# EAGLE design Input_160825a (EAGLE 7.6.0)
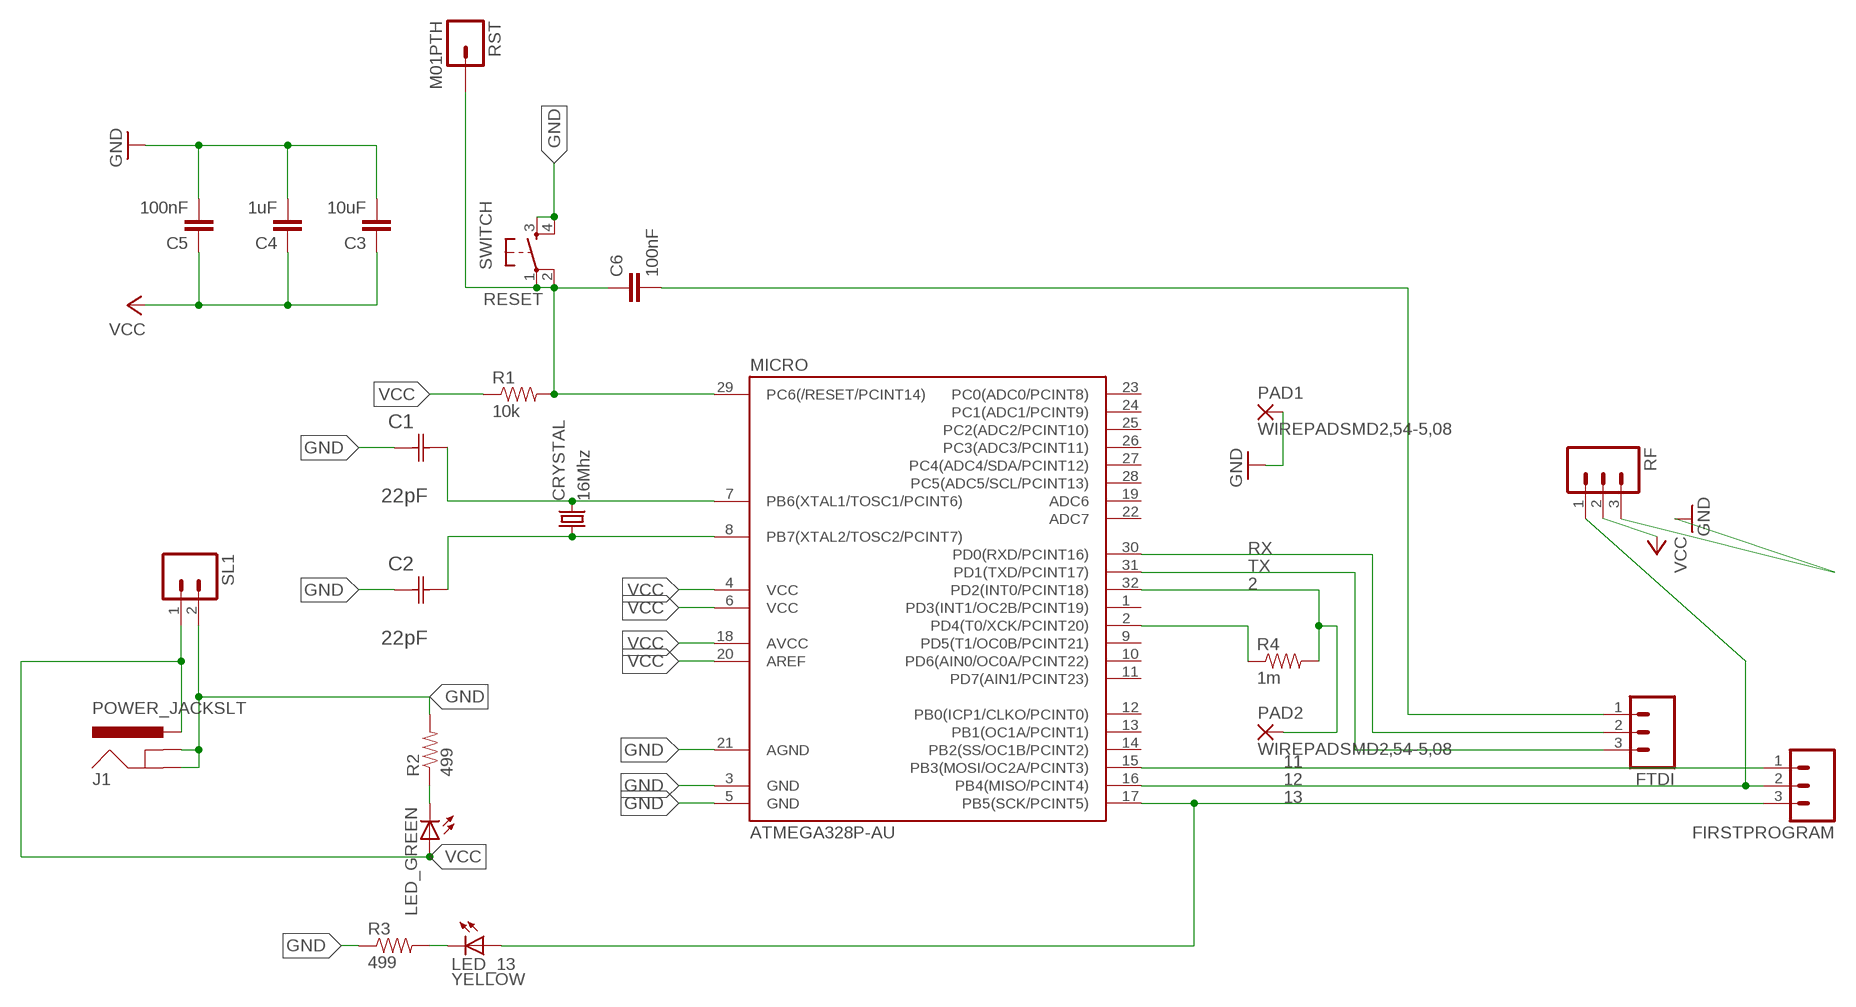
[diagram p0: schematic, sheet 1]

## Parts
C1  22pF  0612ZC225MAT2A  [CAPC3216X178N]
C2  22pF  0612ZC225MAT2A  [CAPC3216X178N]
C3  10uF  CAP1206  [1206]
C4  1uF  CAP1206  [1206]
C5  100nF  CAP1206  [1206]
C6  100nF  CAP1206  [1206]
CRYSTAL  16Mhz  CSM-7X-DU  [CSM-7X-DU]
FIRSTPROGRAM  M03  [03P]
FTDI  M03  [03P]
J1  POWER_JACKSLT  [POWER_JACK_SLOT]
LED_13  YELLOW  LED1206  [1206]
LED_GREEN  LED1206  [1206]
MICRO  ATMEGA328P-AU  ATMEGA48/88/168-AU  [TQFP32-08]
PAD1  WIREPADSMD2,54-5,08  [SMD2,54-5,08]
PAD2  WIREPADSMD2,54-5,08  [SMD2,54-5,08]
R1  10k  RESISTOR1206  [1206]
R2  499  RESISTOR1206  [1206]
R3  499  RESISTOR1206  [1206]
R4  1m  RESISTOR1206  [1206]
RF  M03  [03P]
RST  M01PTH  [1X01]
SL1  M02  [02P]
SWITCH  6MM_SWITCH6MM_SWITCH  [6MM_SWITCH]

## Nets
2: MICRO.32(PD2(INT0/PCINT18)) PAD2.1(P) R4.2
11: FIRSTPROGRAM.1 MICRO.15(PB3(MOSI/OC2A/PCINT3))
12: FIRSTPROGRAM.2 MICRO.16(PB4(MISO/PCINT4)) RF.1
13: FIRSTPROGRAM.3 LED_13.1(A) MICRO.17(PB5(SCK/PCINT5))
GND: C1.1(C1) C2.1(C1) C3.2 C4.2 C5.2 J1.GND@1(GNDBREAK) J1.GND@2(GND) MICRO.3(GND) MICRO.5(GND) MICRO.21(AGND) PAD1.1(P) R2.2 R3.1 RF.3 SL1.2 SWITCH.3(S) SWITCH.4(S1)
N$2: C1.2(C2) CRYSTAL.2 MICRO.7(PB6(XTAL1/TOSC1/PCINT6))
N$3: C6.2 FTDI.1
N$8: MICRO.2(PD4(T0/XCK/PCINT20)) R4.1
N$9: C2.2(C2) CRYSTAL.1 MICRO.8(PB7(XTAL2/TOSC2/PCINT7))
N$26: LED_GREEN.2(C) R2.1
N$27: LED_13.2(C) R3.2
RESET: C6.1 MICRO.29(PC6(/RESET/PCINT14)) R1.2 RST.1 SWITCH.1(P) SWITCH.2(P1)
RX: FTDI.2 MICRO.30(PD0(RXD/PCINT16))
TX: FTDI.3 MICRO.31(PD1(TXD/PCINT17))
VCC: C3.1 C4.1 C5.1 J1.PWR LED_GREEN.1(A) MICRO.4(VCC) MICRO.6(VCC) MICRO.18(AVCC) MICRO.20(AREF) R1.1 RF.2 SL1.1
Unconnected: MICRO.1(PD3(INT1/OC2B/PCINT19)) MICRO.9(PD5(T1/OC0B/PCINT21)) MICRO.10(PD6(AIN0/OC0A/PCINT22)) MICRO.11(PD7(AIN1/PCINT23)) MICRO.12(PB0(ICP1/CLKO/PCINT0)) MICRO.13(PB1(OC1A/PCINT1)) MICRO.14(PB2(SS/OC1B/PCINT2)) MICRO.19(ADC6) MICRO.22(ADC7) MICRO.23(PC0(ADC0/PCINT8)) MICRO.24(PC1(ADC1/PCINT9)) MICRO.25(PC2(ADC2/PCINT10)) MICRO.26(PC3(ADC3/PCINT11)) MICRO.27(PC4(ADC4/SDA/PCINT12)) MICRO.28(PC5(ADC5/SCL/PCINT13))

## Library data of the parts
C1 C2 = AVX_By_element14_Batch_1:0612ZC225MAT2A: Capacitor 1206; MPN: 0612ZC225MAT2A; OC_FARNELL: -; OC_NEWARK: 12N3209; SUPPLIER: AVX; TOLERANCE: ±20%; VALUE: 2.2µF; VOLTAGERATING: 10V
C3-C6 = 01_SparkFun:CAP: Capacitor
CRYSTAL = 01_FAB_Hello:CSM-7X-DU: SMD CRYSTAL; OC_FARNELL: unknown; OC_NEWARK: unknown
FIRSTPROGRAM FTDI RF = con-amp-quick:M03: AMP QUICK CONNECTOR; OC_FARNELL: unknown; OC_NEWARK: unknown
J1 = jib-fab:POWER_JACK: Power Jack This is the standard 5.5mm barrel jack for power. The PTH is the most common, proven, reliable, footprint. The Slot footprint only works if the mill layer is transmitted to the PCB fab house so be warned. Mating wall wart : TOL-00298 (and others); PROD_ID: PRT-00119
LED_13 LED_GREEN = 01_FAB_Hello:LED
MICRO = atmega8:ATMEGA48/88/168
PAD1 PAD2 = wirepad:WIREPAD: Wire PAD connect wire on PCB
R1-R4 = 01_SparkFun:RESISTOR: Resistor
RST = 01_SparkFun:M01: Header 1
SL1 = con-amp-quick:M02: AMP QUICK CONNECTOR; OC_FARNELL: unknown; OC_NEWARK: unknown
SWITCH = 01_FAB_Hello:6MM_SWITCH: OMRON SWITCH

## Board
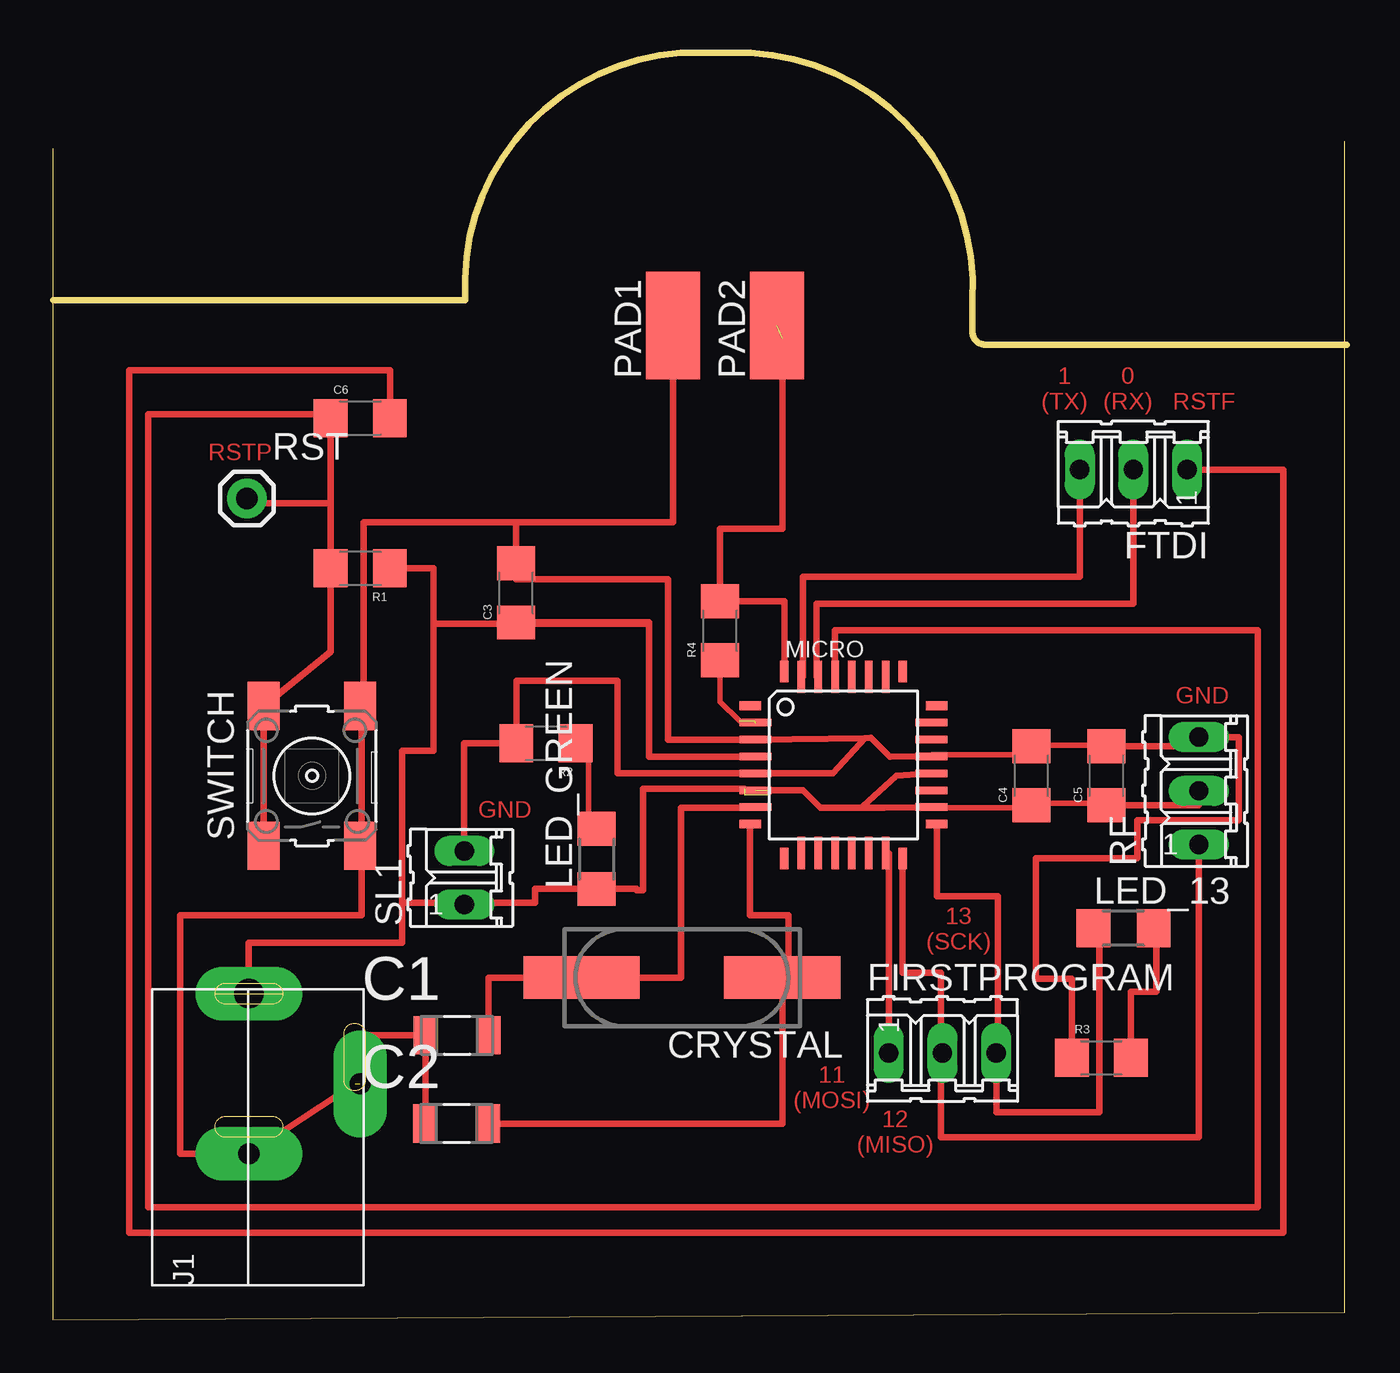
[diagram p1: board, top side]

Size 61.22 x 59.92 mm. Coordinates in mm from the lower left corner, seen from the top.
Outline: 61.12,55.74 61.12,0.35 0,0 0,55.4
Outline: 0.02,48.22 19.52,48.22 arc-90 29.72,59.92 33.02,59.92 arc-90 43.52,48.22 43.52,46.72 arc90 44.12,46.12 61.22,46.12
Copper layers (1*16): Top 0.035mm / dielectric 1.5mm / Bottom 0.035mm
Design rules "default": minimum track width 10mil, minimum drill 24mil, track to track 8mil, track to pad 8mil, pad to pad 8mil, via to via 8mil, smd to smd 8mil, copper to edge 40mil, drill to drill 8mil, minimum pad ring 10mil, minimum via ring 8mil, stop-mask expansion 4mil, vias tented up to drill 0mil, thermal gap 10mil

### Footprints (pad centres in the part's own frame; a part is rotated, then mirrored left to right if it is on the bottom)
CAPC3216X178N = smd 1.118 x 1.803: 1 -1.499,0; 2 1.499,0
1206 = smd 1.6 x 1.8: 1 -1.4,0; 2 1.4,0
CSM-7X-DU = smd 5.5 x 2: 1 -4.75,0; 2 4.75,0
03P = drill 0.914 long: 1 -2.54,0; 2 0,0; 3 2.54,0
POWER_JACK_SLOT = drill 1 pad 2.54 long: GND@1 2.58,6.23; GND@2 7.85,9.53 | drill 1.4 pad 2.54 long: PWR 2.58,13.8
1206' = smd 1.6 x 1.803: 1 -1.422,0; 2 1.422,0
TQFP32-08 = smd 1.016 x 0.406: 1 -4.42,2.8; 8 -4.42,-2.8; 17 4.42,-2.8; 24 4.42,2.8 | smd 1.524 x 0.356: 2 -4.166,2; 3 -4.166,1.2; 4 -4.166,0.4; 5 -4.166,-0.4; 6 -4.166,-1.2; 7 -4.166,-2; 18 4.166,-2; 19 4.166,-1.2; 20 4.166,-0.4; 21 4.166,0.4; 22 4.166,1.2; 23 4.166,2 | smd 0.406 x 1.016: 9 -2.8,-4.42; 16 2.8,-4.42; 25 2.8,4.42; 32 -2.8,4.42 | smd 0.356 x 1.524: 10 -2,-4.166; 11 -1.2,-4.166; 12 -0.4,-4.166; 13 0.4,-4.166; 14 1.2,-4.166; 15 2,-4.166; 26 2,4.166; 27 1.2,4.166; 28 0.4,4.166; 29 -0.4,4.166; 30 -1.2,4.166; 31 -2,4.166
SMD2,54-5,08 = smd 2.54 x 5.08: 1 0,0
1X01 = drill 1.016 pad 1.88: 1 0,0
02P = drill 0.914 long: 1 -1.27,0; 2 1.27,0
6MM_SWITCH = smd 2.286 x 1.524: 1 -3.302,2.286; 2 3.302,2.286; 3 -3.302,-2.286; 4 3.302,-2.286

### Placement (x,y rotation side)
C1  19.12,13.45 0 top
C2  19.1,9.28 0 top
C3  21.91,34.38 90 top
C4  46.3,25.73 90 top
C5  49.85,25.73 90 top
C6  14.55,42.65 0 top
CRYSTAL  29.76,16.18 180 top
FIRSTPROGRAM  42.09,12.62 0 top
FTDI  51.12,40.21 180 top
J1  6.7,1.63 0 top
LED_13  YELLOW  [1206']  50.66,18.52 0 top
LED_GREEN  [1206']  25.72,21.8 90 top
MICRO  37.41,26.24 0 top
PAD1  29.35,47.02 0 top
PAD2  34.26,47.02 0 top
R1  14.55,35.54 180 top
R2  23.33,27.26 180 top
R3  49.61,12.4 0 top
R4  31.56,32.59 90 top
RF  54.22,25.02 90 top
RST  9.19,38.84 0 top
SL1  19.46,20.91 90 top
SWITCH  12.26,25.72 90 top

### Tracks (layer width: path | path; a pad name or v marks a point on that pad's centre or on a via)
2  (1 unrouted)
  Top 0.305: MICRO.32 34.61,33.99 R4.2 31.56,37.42 34.52,37.42 34.52,46.42
11
  Top 0.305: MICRO.15 39.55,22.08 FIRSTPROGRAM.1
12
  Top 0.305: MICRO.16 40.21,16.42 42.02,16.42 42.02,13.12 42.02,12.62 | 42.02,12.62 FIRSTPROGRAM.2 | RF.1 54.22,8.62 42.02,8.62 42.02,12.62
13
  Top 0.305: 41.72,23.44 MICRO.17 41.83,20.02 44.72,20.02 44.72,12.62 FIRSTPROGRAM.3 44.63,9.82 49.52,9.82 49.52,18.52 LED_13.1
GND  (1 unrouted)
  Top 0.254: MICRO.21 41.62,26.73 45.74,26.73 C4.2 46.42,27.18 49.85,27.18 C5.2
  Top 0.305: MICRO.5 | MICRO.21 39.62,26.62 38.72,27.52 38.42,27.5 | 45.8,26.64 arc90 C4.2 | C5.2 53.42,27.13 53.42,27.22 54.22,27.22 RF.3 56.12,27.56 56.12,23.62 51.32,23.62 51.32,21.82 46.52,21.82 46.52,16.12 48.21,16.12 R3.1 | 38.42,27.5 MICRO.3 29.12,27.44 29.12,35.02 21.91,35.02 C3.2 21.91,37.72 | MICRO.5 36.92,25.84 38.42,27.5 | SWITCH.3 14.6,22.42 | C2.1 17.63,9.28 C1.1 14.6,13.45 14.3,11.16 J1.GND@1 6.02,7.86 6.02,19.12 14.6,19.12 14.6,22.42 | 14.6,22.42 14.6,28.42 | 14.6,28.42 14.6,29.03 SWITCH.4 | SL1.2 19.46,27.26 R2.2 21.93,30.22 26.72,30.22 26.72,25.84 MICRO.5 | 21.91,37.72 14.72,37.72 14.72,28.42 14.6,28.42 | 21.91,37.72 29.35,37.72 PAD1.1
N$2
  Top 0.305: C1.2 20.62,16.18 CRYSTAL.2 29.72,16.18 29.72,24.22 33.24,24.22 MICRO.7
N$3
  Top 0.305: C6.2 15.95,44.92 3.62,44.92 3.62,4.12 58.22,4.12 58.22,40.21 FTDI.1
N$8  (2 unrouted)
  Top 0.254: 32.48,28.33 31.56,29.24 R4.1
N$9
  Top 0.305: MICRO.8 32.99,19.12 34.82,19.12 34.82,16.18 CRYSTAL.1 34.51,9.28 C2.2
N$26
  Top 0.254: R2.1 25.33,26.95 25.33,23.98 25.85,23.3 LED_GREEN.2
N$27
  Top 0.305: R3.2 51.01,15.52 52.22,15.52 52.22,18.52 LED_13.2
RESET
  Top 0.305: SWITCH.1 SWITCH.2 13.15,31.6 R1.2 13.15,38.62 | 13.15,38.62 C6.1 12.92,42.65 12.92,42.82 4.52,42.82 4.52,5.32 57.02,5.32 57.02,32.62 37.01,32.62 MICRO.29 | RST.1 9.19,38.62 13.15,38.62
RX
  Top 0.305: FTDI.2 51.12,33.86 36.14,33.86 36.14,30.41 MICRO.30
TX
  Top 0.305: FTDI.3 48.58,35.13 35.5,35.13 35.5,30.41 MICRO.31
VCC  (4 unrouted)
  Top 0.254: MICRO.18 41.62,24.21 46.19,24.21 C4.1 46.42,24.44 49.85,24.44 C5.1
  Top 0.305: MICRO.18 39.32,24.23 | C5.1 54.22,24.34 RF.2 | 39.32,24.23 38.72,24.22 38.33,24.28 39.92,25.72 MICRO.20 | MICRO.6 35.5,25.04 36.32,24.22 39.31,24.22 39.32,24.23 | 32.72,25.12 27.92,25.12 27.92,20.32 27.62,20.32 27.62,20.38 LED_GREEN.1 22.82,20.38 22.82,19.72 19.46,19.72 | C3.1 28.22,32.98 28.22,32.92 | MICRO.4 33.24,26.62 28.22,26.62 28.22,32.92 | 16.52,19.72 16.52,26.92 18.02,26.92 18.02,32.92 | 16.52,19.72 19.46,19.72 | 19.46,19.72 SL1.1 | R1.1 18.02,35.54 18.02,32.92 | 28.22,32.92 18.02,32.92 | 16.52,19.72 16.52,17.83 9.28,17.83 J1.PWR

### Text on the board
Top: 1 / (TX) | 0 / (RX) | RSTF | RSTP | GND | GND | 13 / (SCK) | 11 / (MOSI) | 12 / (MISO)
